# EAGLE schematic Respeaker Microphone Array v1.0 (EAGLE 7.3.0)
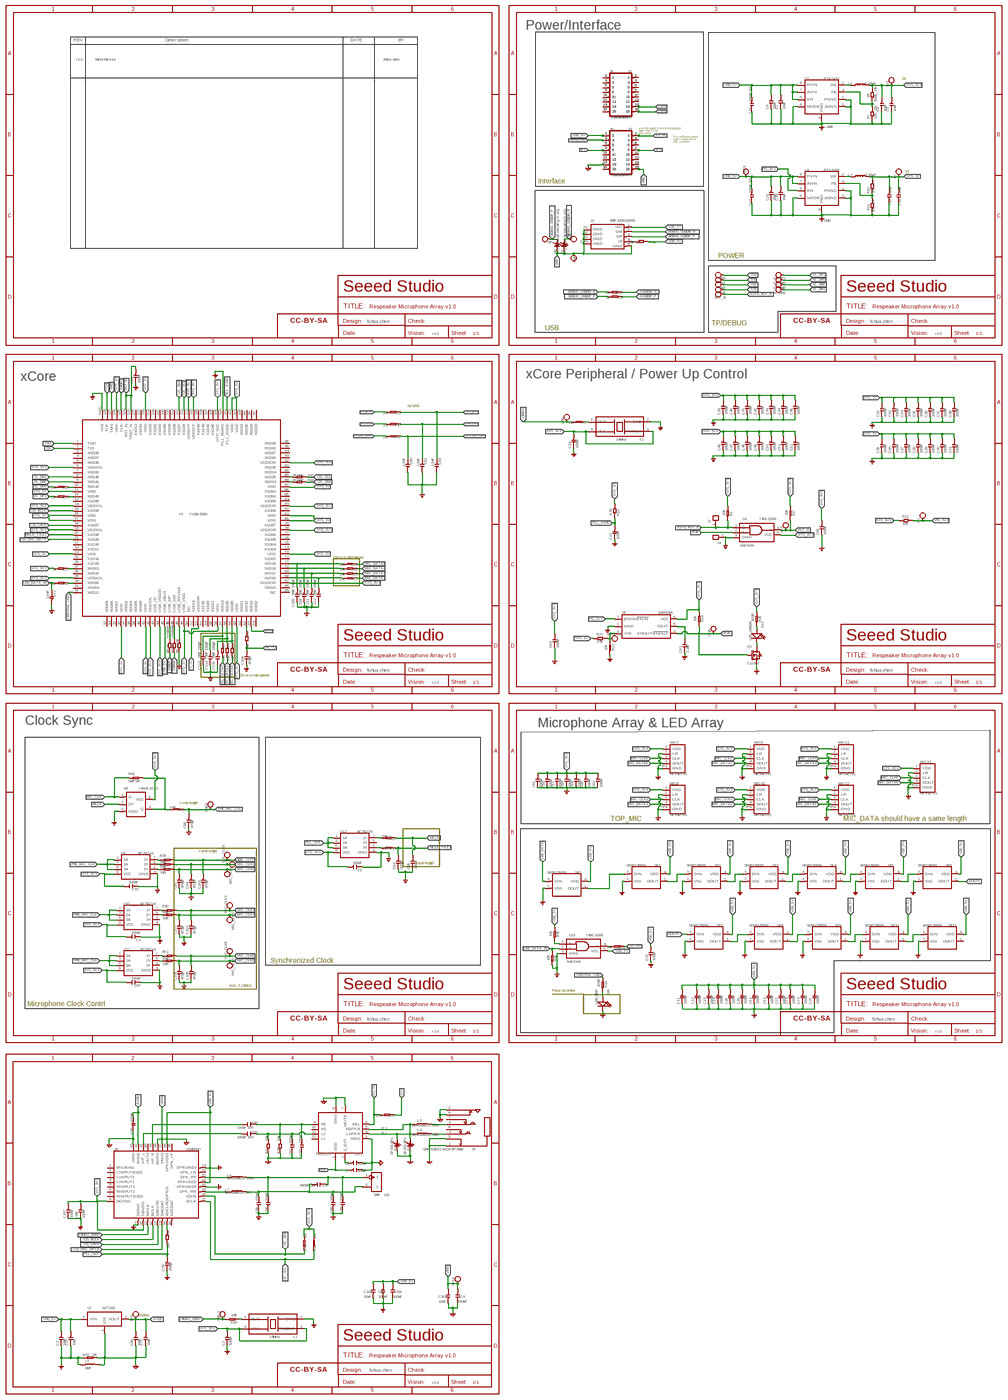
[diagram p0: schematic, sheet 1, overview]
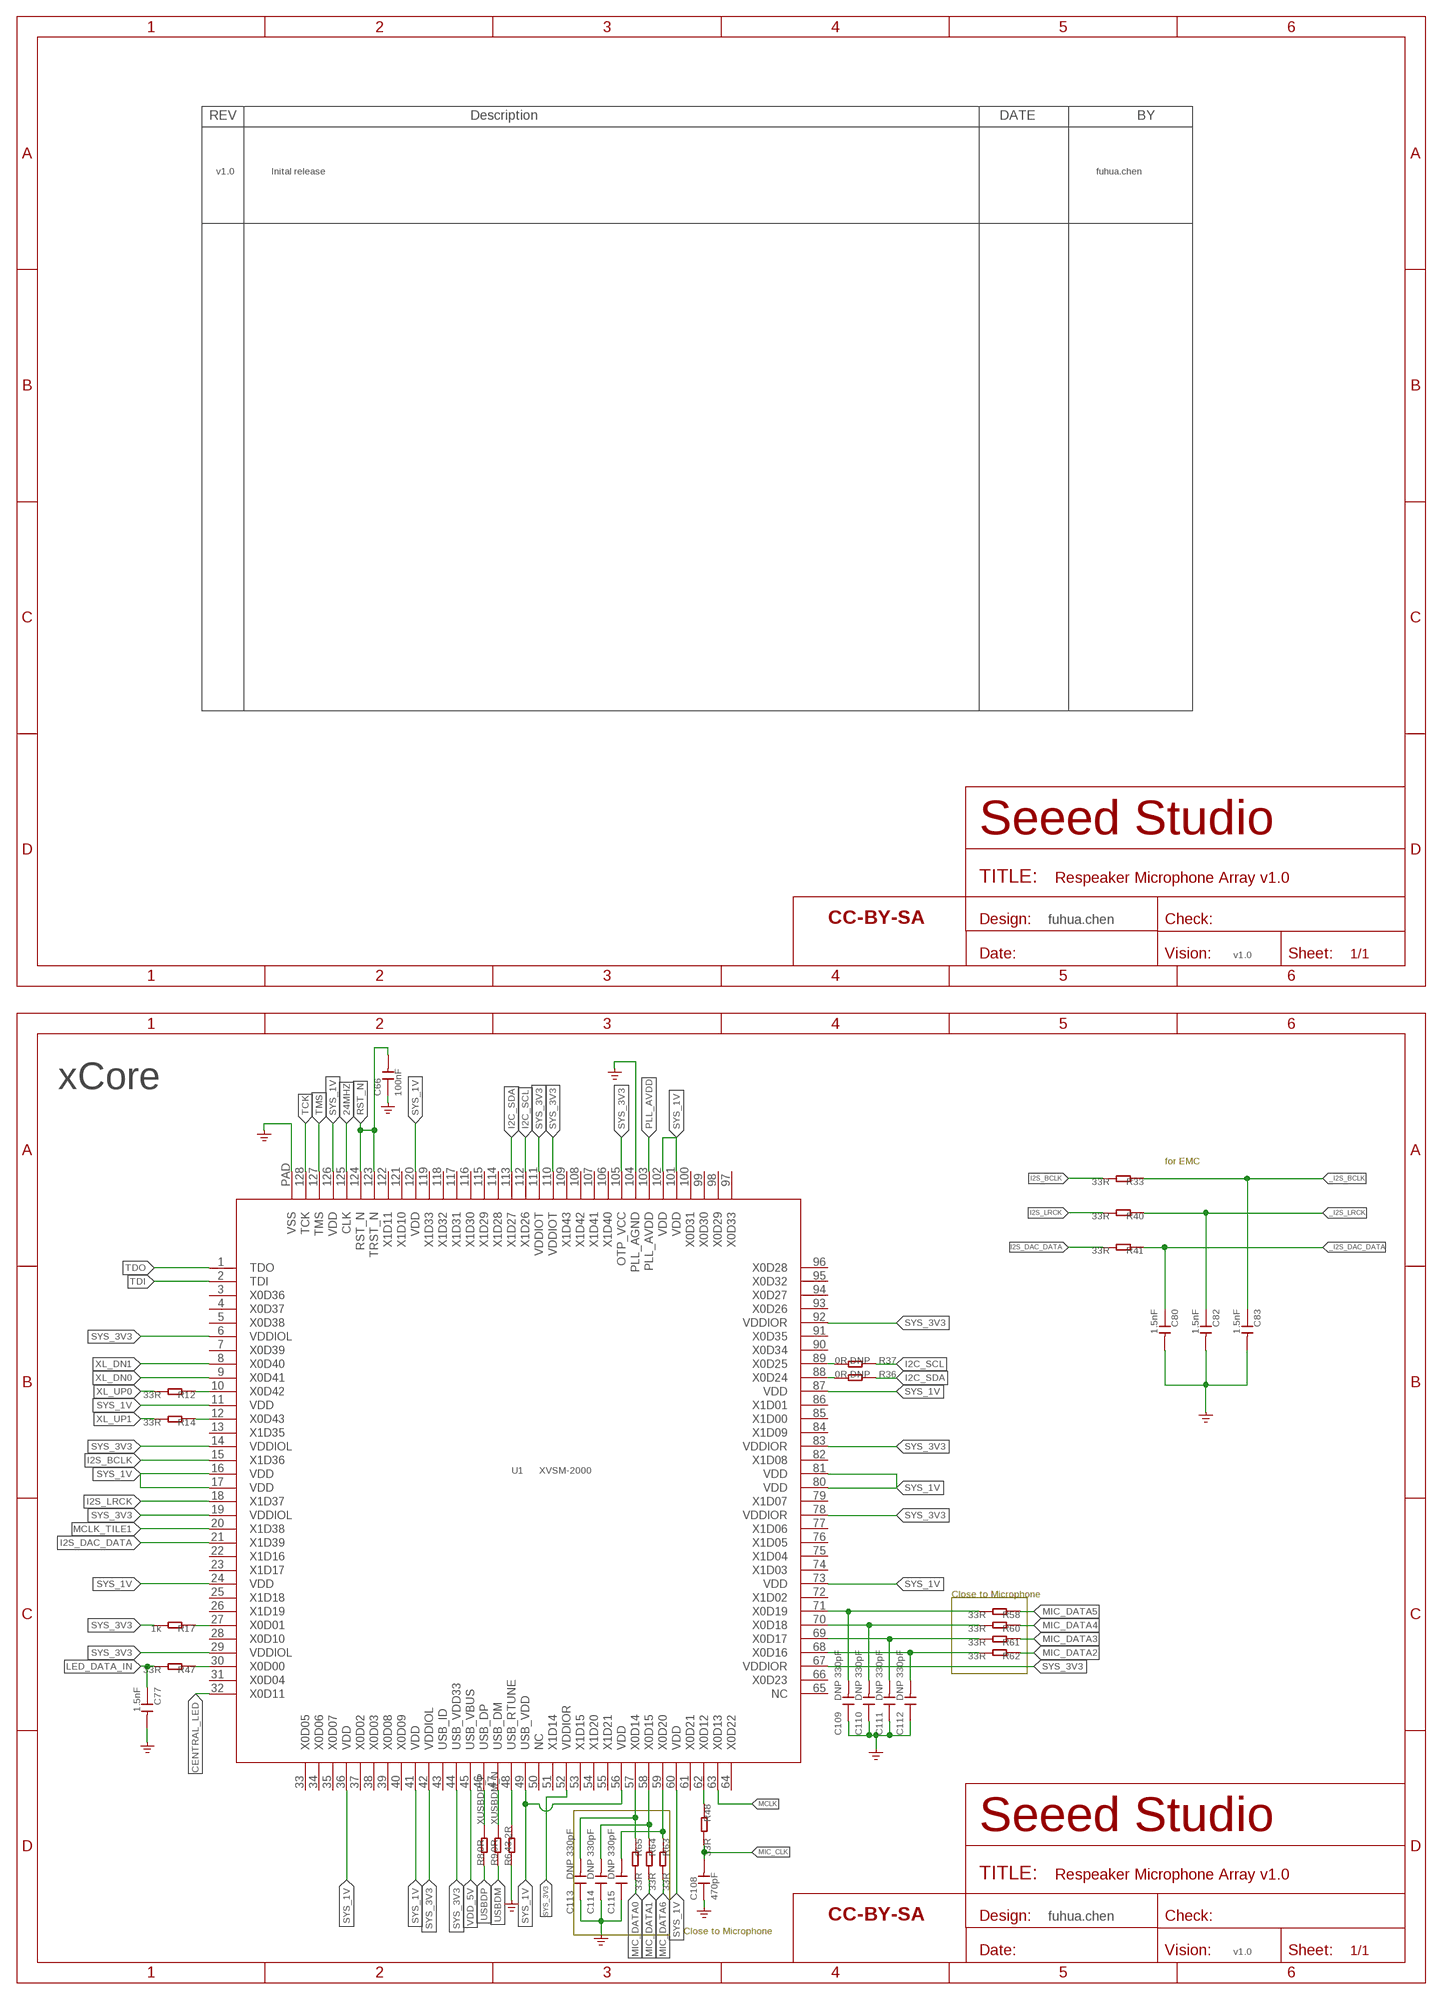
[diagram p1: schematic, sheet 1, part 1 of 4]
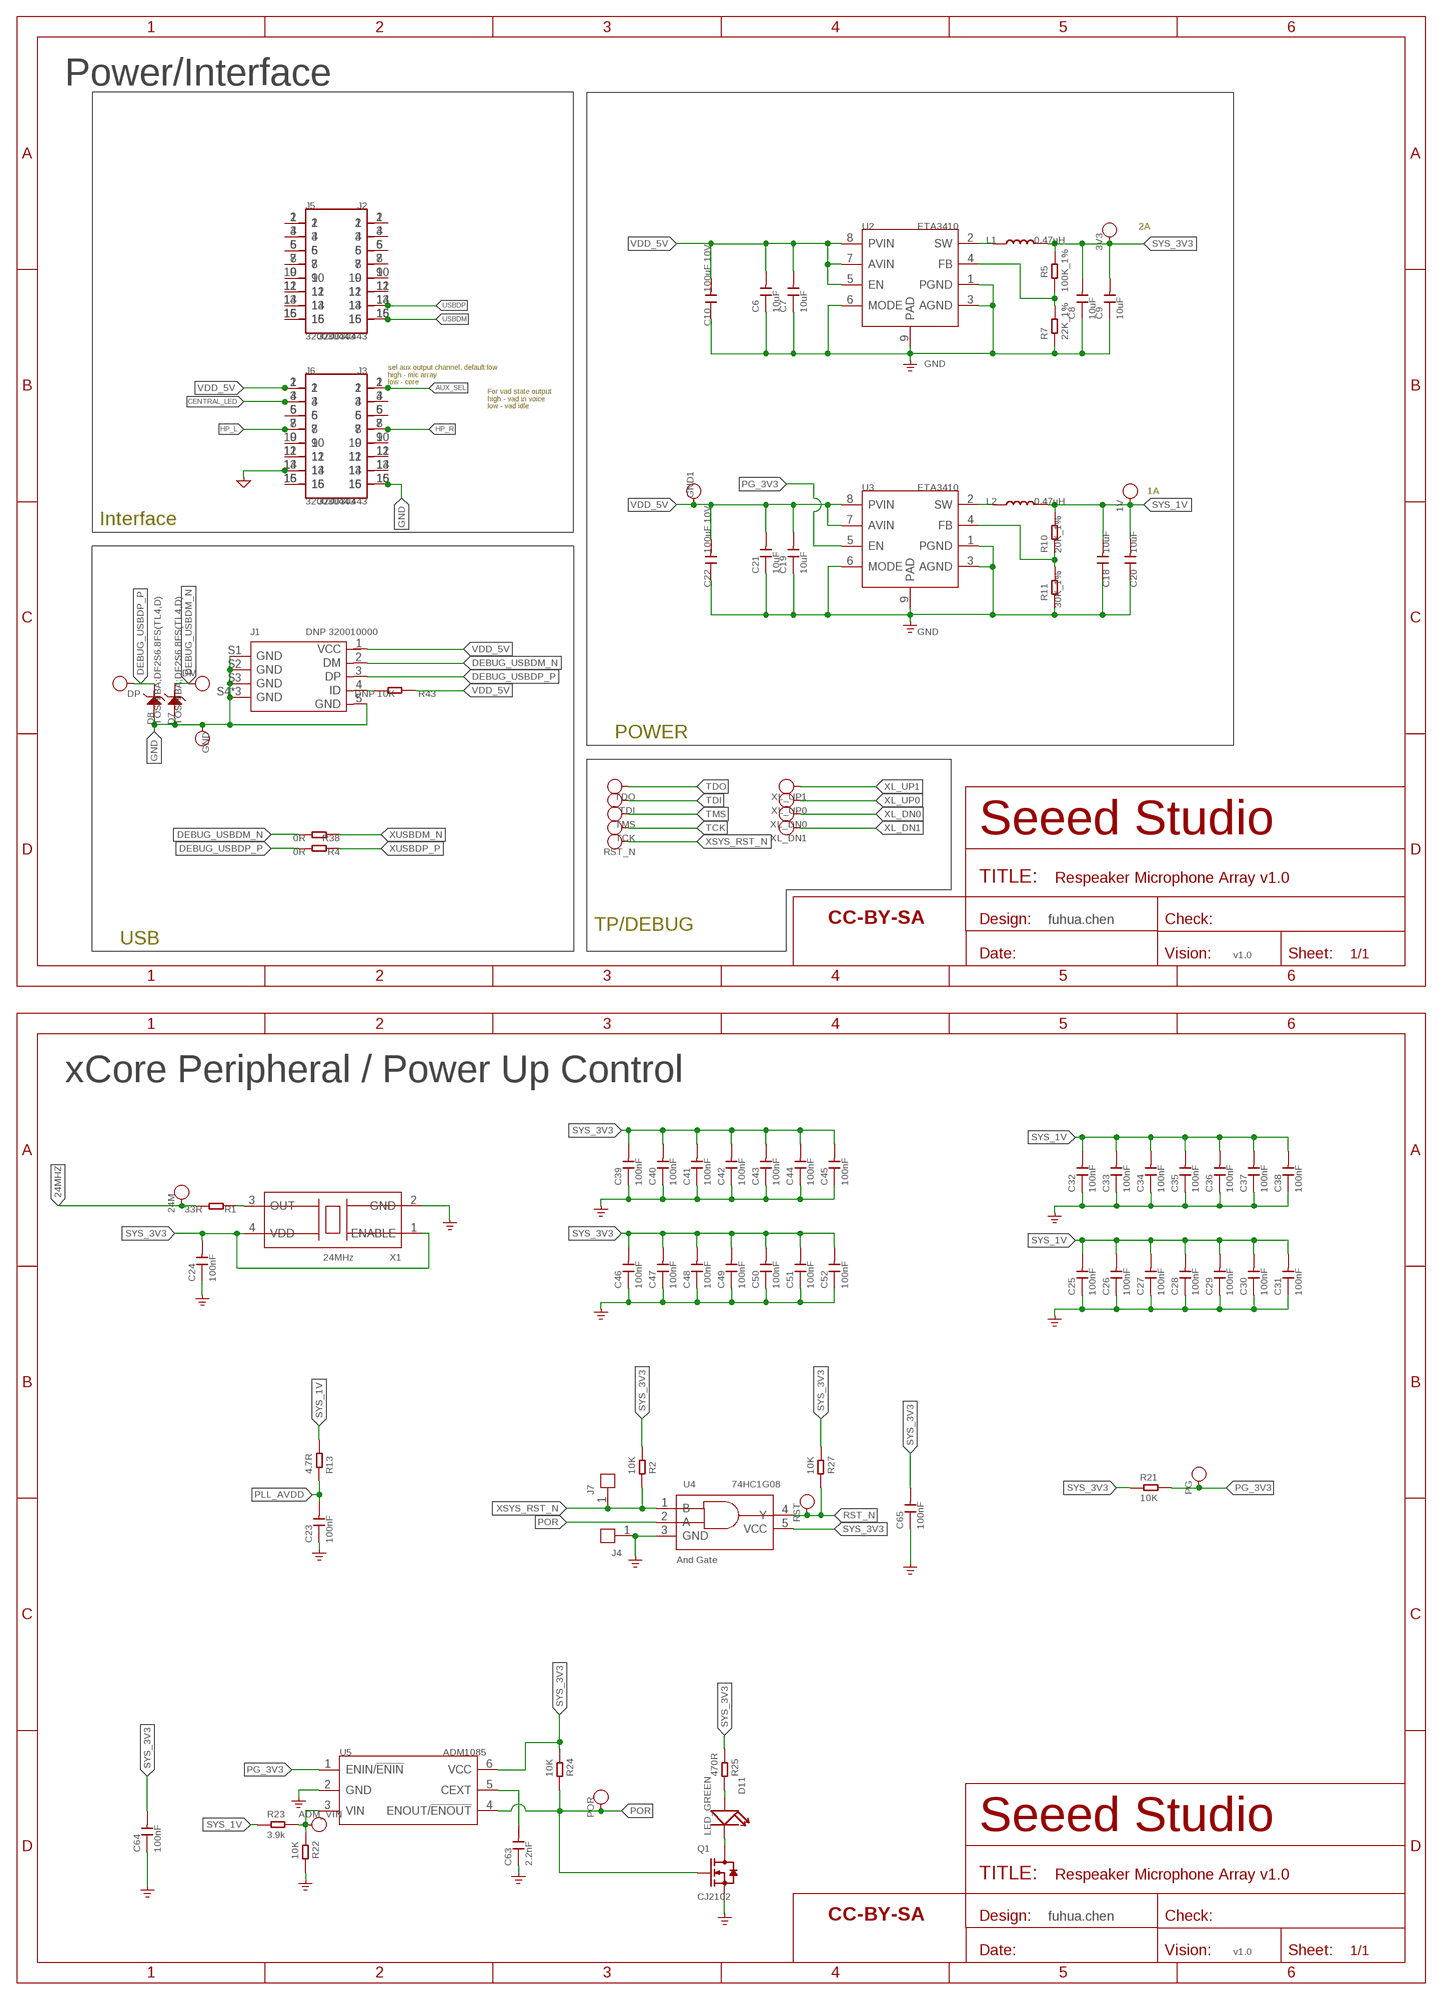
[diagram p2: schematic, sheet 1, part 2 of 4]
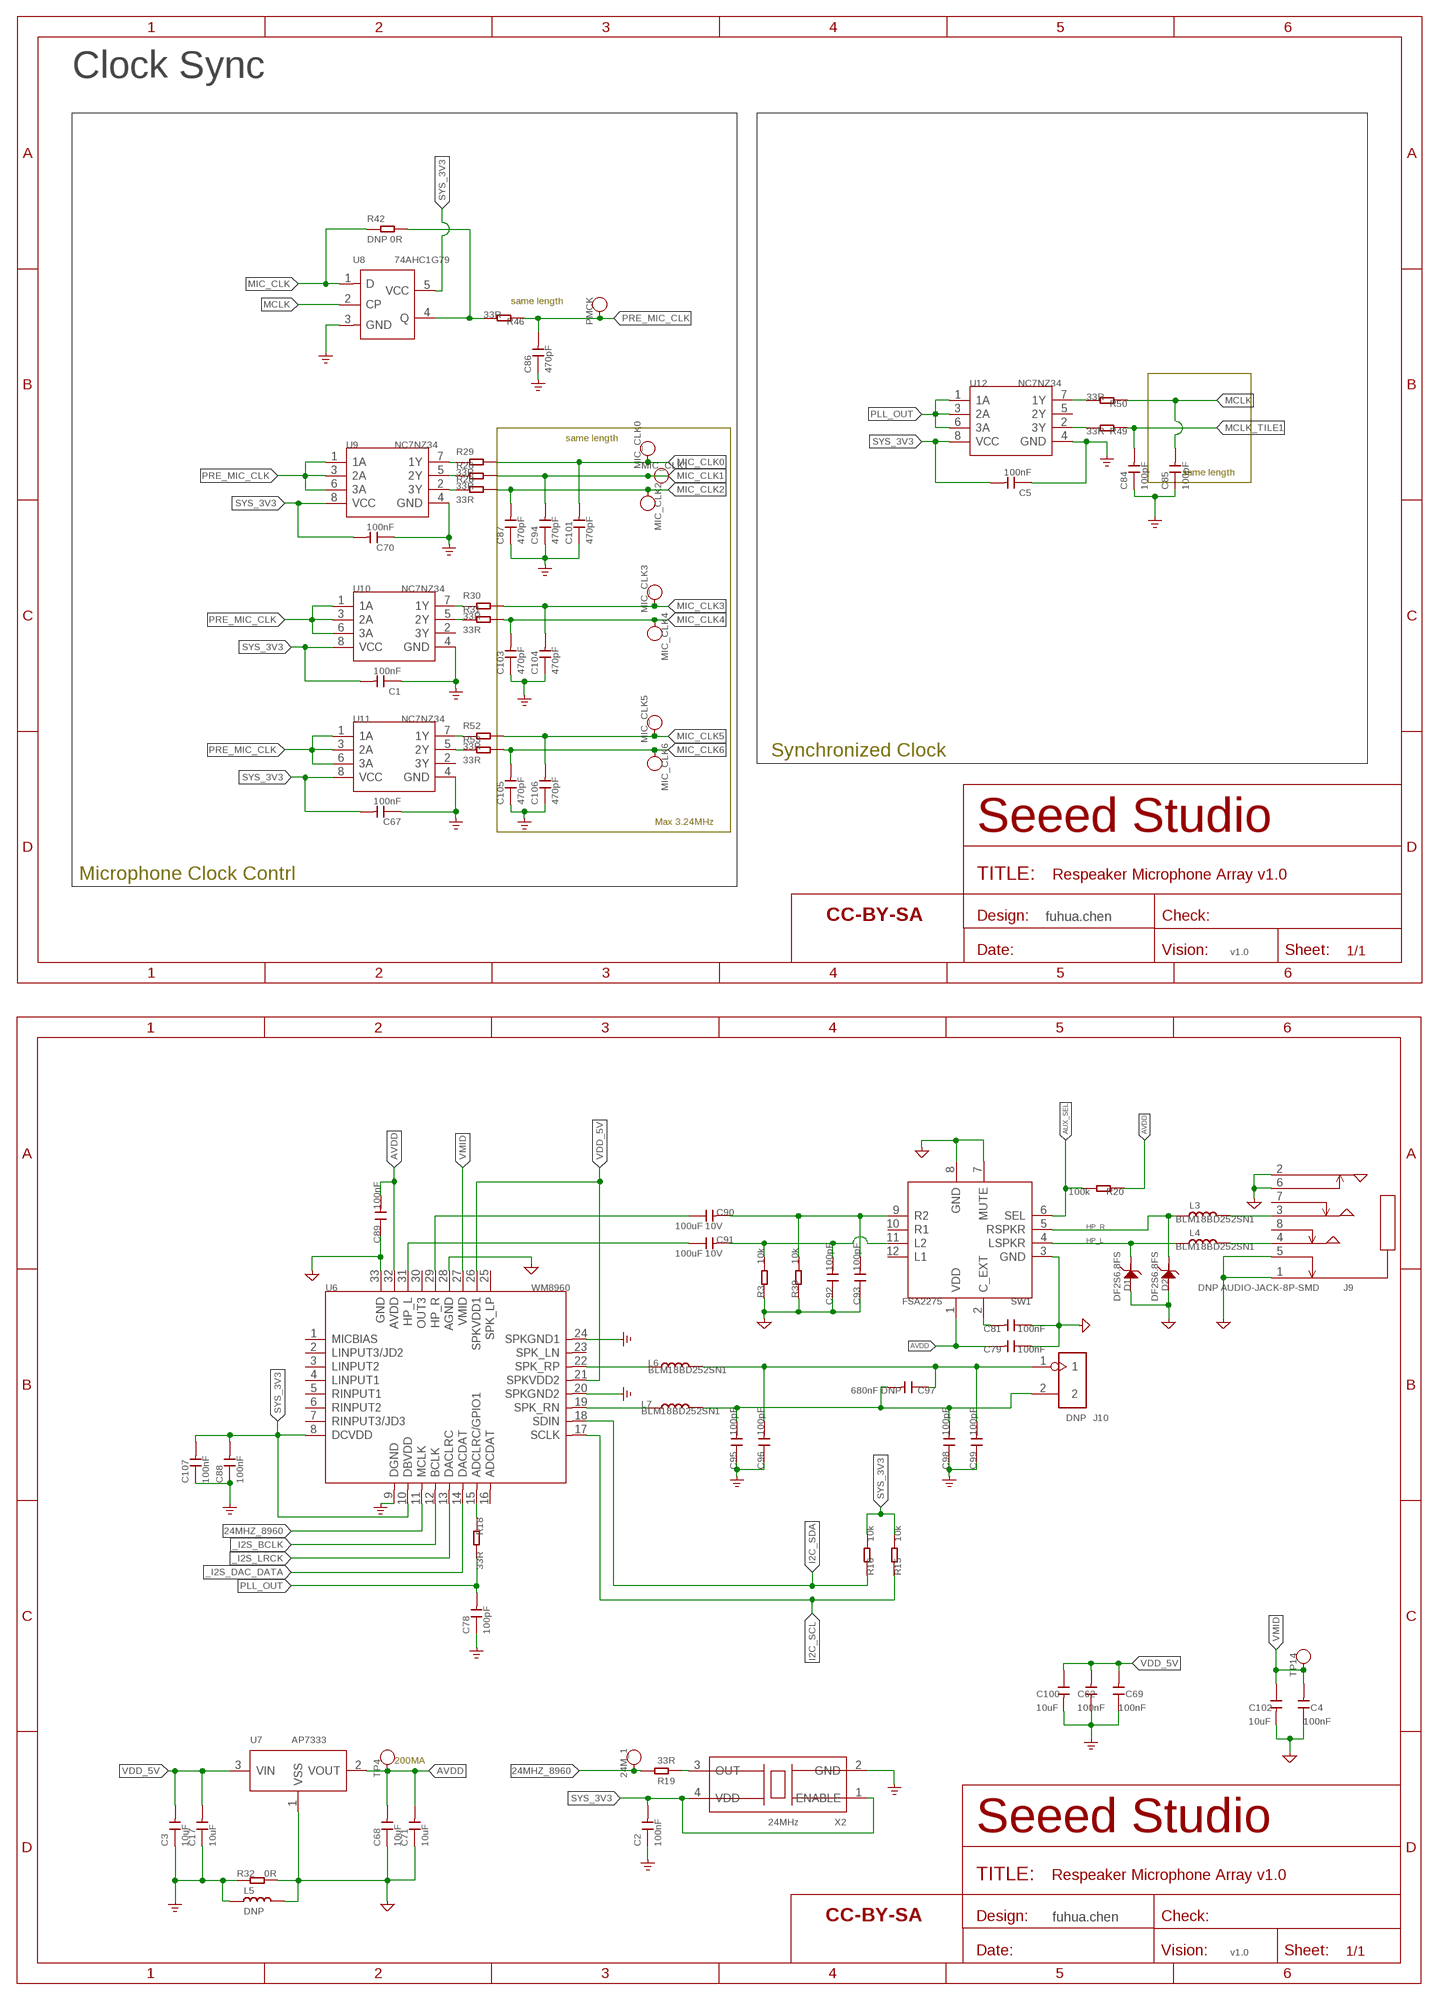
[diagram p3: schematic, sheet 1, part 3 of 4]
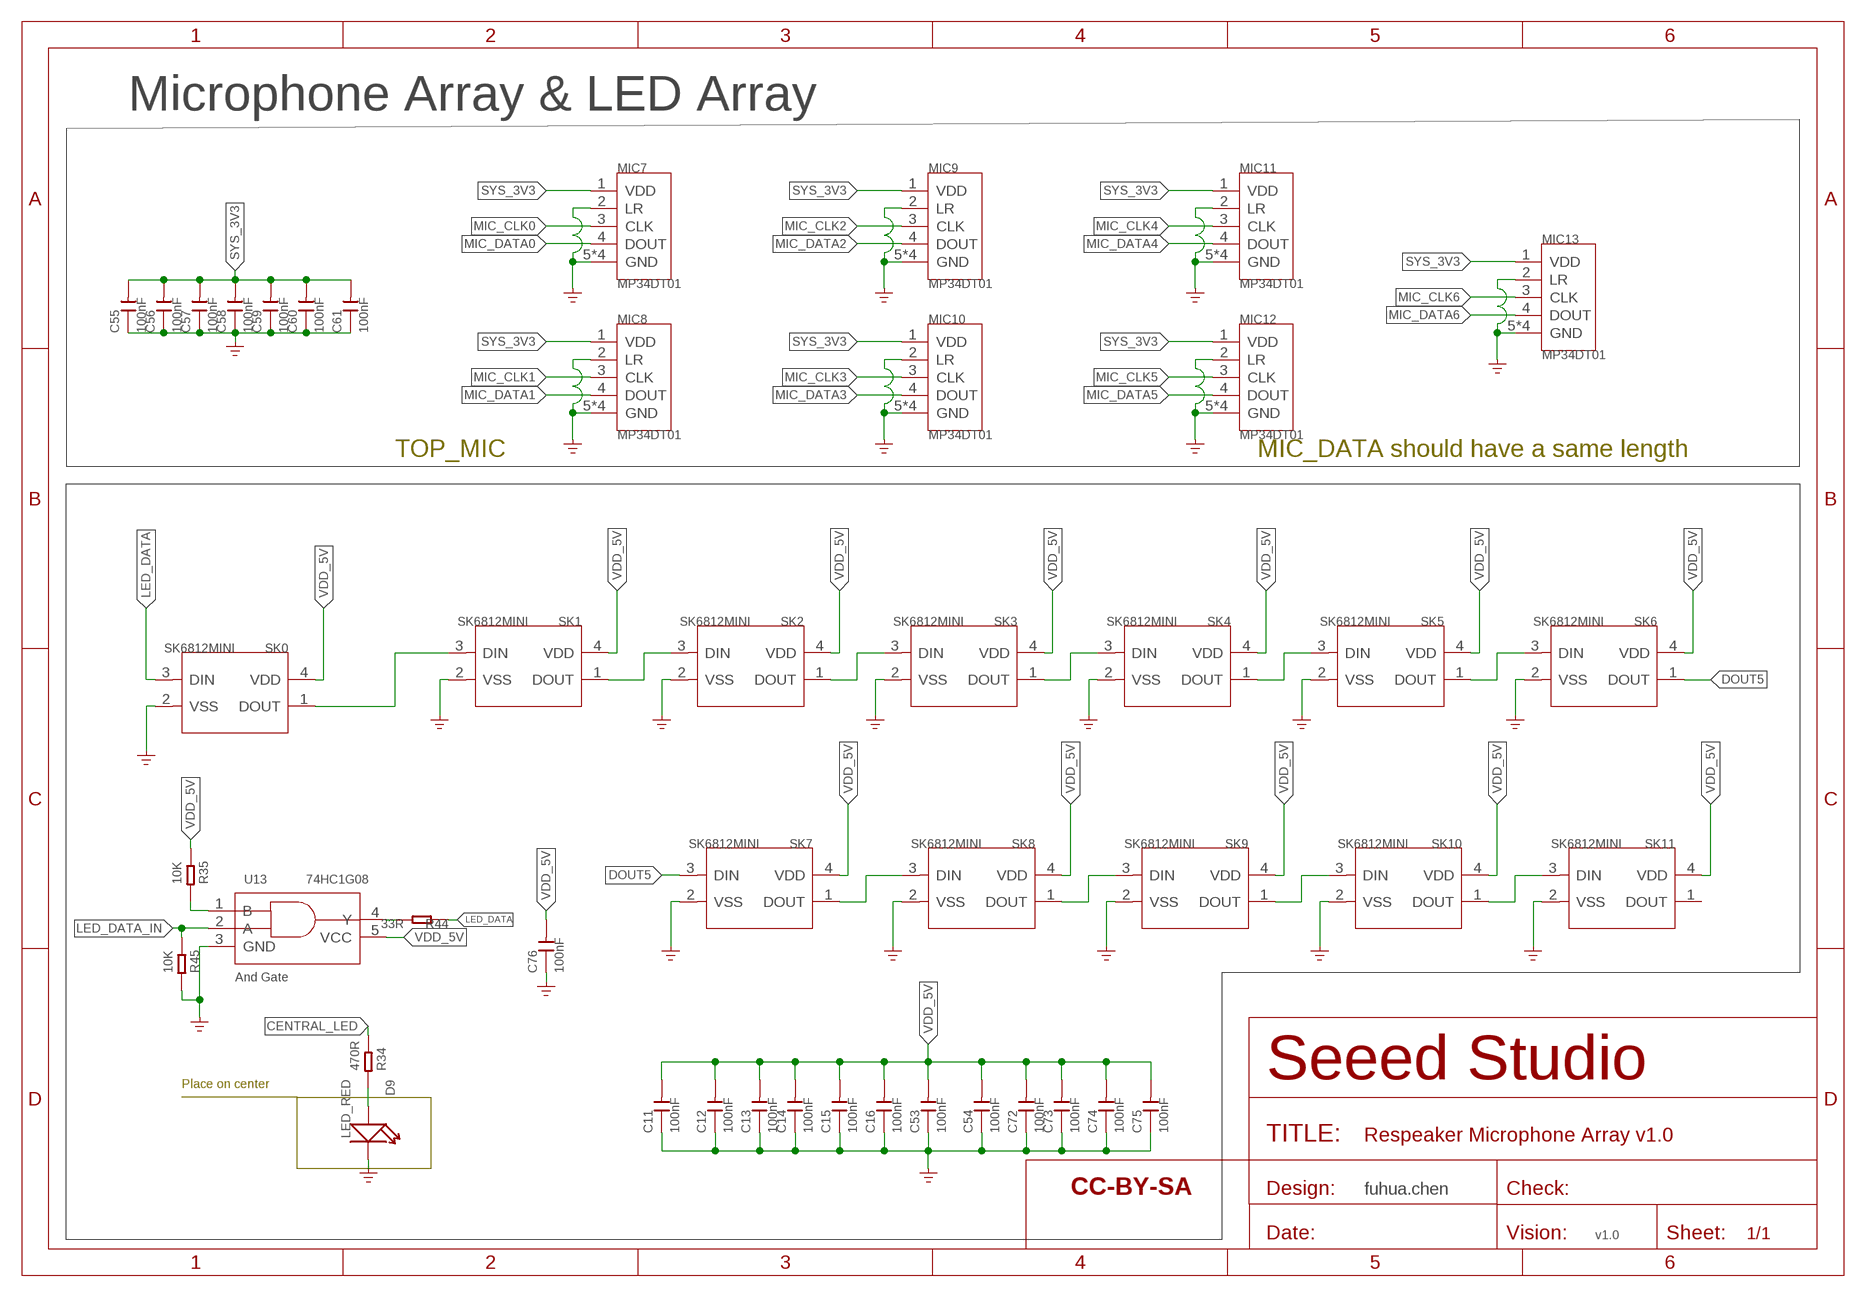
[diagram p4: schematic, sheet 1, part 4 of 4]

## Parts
1V  TEST-POINT'4545'  [TP-D45MIL]
3V3  TEST-POINT'4545'  [TP-D45MIL]
24M  TEST-POINT'4545'  [TP-D45MIL]
24M_1  TEST-POINT'4545'  [TP-D45MIL]
ADM_VIN  TEST-POINT'4545'  [TP-D45MIL]
C1  100nF  CAP-0402  [C0402]
C2  100nF  CAP-0402  [C0402]
C3  10uF  CAP-0603  [C0603]
C4  100nF  CAP-0402  [C0402]
C5  100nF  CAP-0402  [C0402]
C6  10uF  CAP-0603  [C0603]
C7  10uF  CAP-0603  [C0603]
C8  10uF  CAP-0603  [C0603]
C9  10uF  CAP-0603  [C0603]
C10  100uF 10V  CAP-1206  [C1206]
C11  100nF  CAP-0402  [C0402]
C12  100nF  CAP-0402  [C0402]
C13  100nF  CAP-0402  [C0402]
C14  100nF  CAP-0402  [C0402]
C15  100nF  CAP-0402  [C0402]
C16  100nF  CAP-0402  [C0402]
C17  10uF  CAP-0603  [C0603]
C18  10uF  CAP-0603  [C0603]
C19  10uF  CAP-0603  [C0603]
C20  10uF  CAP-0603  [C0603]
C21  10uF  CAP-0603  [C0603]
C22  100uF 10V  CAP-1206  [C1206]
C23  100nF  CAP-0402  [C0402]
C24  100nF  CAP-0402  [C0402]
C25  100nF  CAP-0402  [C0402]
C26  100nF  CAP-0402  [C0402]
C27  100nF  CAP-0402  [C0402]
C28  100nF  CAP-0402  [C0402]
C29  100nF  CAP-0402  [C0402]
C30  100nF  CAP-0402  [C0402]
C31  100nF  CAP-0402  [C0402]
C32  100nF  CAP-0402  [C0402]
C33  100nF  CAP-0402  [C0402]
C34  100nF  CAP-0402  [C0402]
C35  100nF  CAP-0402  [C0402]
C36  100nF  CAP-0402  [C0402]
C37  100nF  CAP-0402  [C0402]
C38  100nF  CAP-0402  [C0402]
C39  100nF  CAP-0402  [C0402]
C40  100nF  CAP-0402  [C0402]
C41  100nF  CAP-0402  [C0402]
C42  100nF  CAP-0402  [C0402]
C43  100nF  CAP-0402  [C0402]
C44  100nF  CAP-0402  [C0402]
C45  100nF  CAP-0402  [C0402]
C46  100nF  CAP-0402  [C0402]
C47  100nF  CAP-0402  [C0402]
C48  100nF  CAP-0402  [C0402]
C49  100nF  CAP-0402  [C0402]
C50  100nF  CAP-0402  [C0402]
C51  100nF  CAP-0402  [C0402]
C52  100nF  CAP-0402  [C0402]
C53  100nF  CAP-0402  [C0402]
C54  100nF  CAP-0402  [C0402]
C55  100nF  CAP-0402  [C0402]
C56  100nF  CAP-0402  [C0402]
C57  100nF  CAP-0402  [C0402]
C58  100nF  CAP-0402  [C0402]
C59  100nF  CAP-0402  [C0402]
C60  100nF  CAP-0402  [C0402]
C61  100nF  CAP-0402  [C0402]
C62  100nF  CAP-0402  [C0402]
C63  2.2nF  CAP-0402  [C0402]
C64  100nF  CAP-0402  [C0402]
C65  100nF  CAP-0402  [C0402]
C66  100nF  CAP-0402  [C0402]
C67  100nF  CAP-0402  [C0402]
C68  10uF  CAP-0603  [C0603]
C69  100nF  CAP-0402  [C0402]
C70  100nF  CAP-0402  [C0402]
C71  10uF  CAP-0603  [C0603]
C72  100nF  CAP-0402  [C0402]
C73  100nF  CAP-0402  [C0402]
C74  100nF  CAP-0402  [C0402]
C75  100nF  CAP-0402  [C0402]
C76  100nF  CAP-0402  [C0402]
C77  1.5nF  CAP-0402  [C0402]
C78  100pF  CAP-0402  [C0402]
C79  100nF  CAP-0402  [C0402]
C80  1.5nF  CAP-0402  [C0402]
C81  100nF  CAP-0402  [C0402]
C82  1.5nF  CAP-0402  [C0402]
C83  1.5nF  CAP-0402  [C0402]
C84  100pF  CAP-0402  [C0402]
C85  100pF  CAP-0402  [C0402]
C86  470pF  CAP-0402  [C0402]
C87  470pF  CAP-0402  [C0402]
C88  100nF  CAP-0402  [C0402]
C89  100nF  CAP-0402  [C0402]
C90  100uF 10V  CAP-1206  [C1206]
C91  100uF 10V  CAP-1206  [C1206]
C92  100pF  CAP-0402  [C0402]
C93  100pF  CAP-0402  [C0402]
C94  470pF  CAP-0402  [C0402]
C95  100pF  CAP-0402  [C0402]
C96  100pF  CAP-0402  [C0402]
C97  680nF DNP  CAP-0402  [C0402]
C98  100pF  CAP-0402  [C0402]
C99  100pF  CAP-0402  [C0402]
C100  10uF  CAP-0603  [C0603]
C101  470pF  CAP-0402  [C0402]
C102  10uF  CAP-0603  [C0603]
C103  470pF  CAP-0402  [C0402]
C104  470pF  CAP-0402  [C0402]
C105  470pF  CAP-0402  [C0402]
C106  470pF  CAP-0402  [C0402]
C107  100nF  CAP-0402  [C0402]
C108  470pF  CAP-0402  [C0402]
C109  DNP 330pF  CAP-0402  [C0402]
C110  DNP 330pF  CAP-0402  [C0402]
C111  DNP 330pF  CAP-0402  [C0402]
C112  DNP 330pF  CAP-0402  [C0402]
C113  DNP 330pF  CAP-0402  [C0402]
C114  DNP 330pF  CAP-0402  [C0402]
C115  DNP 330pF  CAP-0402  [C0402]
D1  DF2S6.8FS  D-ESD-2P'DF2S6.8FS'  [SOD-923]
D2  DF2S6.8FS  D-ESD-2P'DF2S6.8FS'  [SOD-923]
D7  TOSHIBA;DF2S6.8FS(TL4,D)  D-ESD-2P'DF2S6.8FS'  [SOD-923]
D8  TOSHIBA;DF2S6.8FS(TL4,D)  D-ESD-2P'DF2S6.8FS'  [SOD-923]
D9  LED_RED  LED-0402  [LED-0402]
D11  LED_GREEN  LED-0402  [LED-0402]
DM  TEST-POINT'4545'  [TP-D45MIL]
DP  TEST-POINT'4545'  [TP-D45MIL]
FR1  SEEEDSTUDIO-OPEN-SCH-FRAME  [SEEEDSTUDIO-PCB-FRAME]
FR2  SEEEDSTUDIO-OPEN-SCH-FRAME  [SEEEDSTUDIO-PCB-FRAME]
FR3  SEEEDSTUDIO-OPEN-SCH-FRAME  [SEEEDSTUDIO-PCB-FRAME]
FR4  SEEEDSTUDIO-OPEN-SCH-FRAME  [SEEEDSTUDIO-PCB-FRAME]
FR5  SEEEDSTUDIO-OPEN-SCH-FRAME  [SEEEDSTUDIO-PCB-FRAME]
FR7  SEEEDSTUDIO-OPEN-SCH-FRAME  [SEEEDSTUDIO-PCB-FRAME]
FR8  SEEEDSTUDIO-OPEN-SCH-FRAME  [SEEEDSTUDIO-PCB-FRAME]
GND  TEST-POINT'4545'  [TP-D45MIL]
GND1  TEST-POINT'4545'  [TP-D45MIL]
J1  DNP 320010000  MICRO-USB5+4P'5+4P'  [MICRO-USB5+4P-SMD-0.65-B]
J2  320030443  HEADER-2X8P-SMD-2.0  [H2X8-SMD-2.0]
J3  320030443  HEADER-2X8P-SMD-2.0  [H2X8-SMD-2.0]
J4  HEADER-1P'20'  [1P-40/25MIL]
J5  320030443  HEADER-2X8P-SMD-2.0  [H2X8-SMD-2.0]
J6  320030443  HEADER-2X8P-SMD-2.0  [H2X8-SMD-2.0]
J7  HEADER-1P'20'  [1P-40/25MIL]
J9  DNP AUDIO-JACK-8P-SMD  AUDIO-JACK-8P-SMD'PJ-393'  [AUDIO8P-SMD-3.5-14.5X6.1X4.0MM]
J10  DNP  HEADER-2P-65/35MIL  [H2-2.54]
L1  0.47uH  L-MPM201610SR33_T  [L201610]
L2  0.47uH  L-MPM201610SR33_T  [L201610]
L3  BLM18BD252SN1  INDUCTOR/FERRITE-BEAD'0603'  [L0603]
L4  BLM18BD252SN1  INDUCTOR/FERRITE-BEAD'0603'  [L0603]
L5  DNP  INDUCTOR/FERRITE-BEAD'0603'  [L0603]
L6  BLM18BD252SN1  INDUCTOR/FERRITE-BEAD'0603'  [L0603]
L7  BLM18BD252SN1  INDUCTOR/FERRITE-BEAD'0603'  [L0603]
MIC7  MP34DT01  MICROPHONE-MP34DT01  [HCLGA5P-3X4X1MM]
MIC8  MP34DT01  MICROPHONE-MP34DT01  [HCLGA5P-3X4X1MM]
MIC9  MP34DT01  MICROPHONE-MP34DT01  [HCLGA5P-3X4X1MM]
MIC10  MP34DT01  MICROPHONE-MP34DT01  [HCLGA5P-3X4X1MM]
MIC11  MP34DT01  MICROPHONE-MP34DT01  [HCLGA5P-3X4X1MM]
MIC12  MP34DT01  MICROPHONE-MP34DT01  [HCLGA5P-3X4X1MM]
MIC13  MP34DT01  MICROPHONE-MP34DT01  [HCLGA5P-3X4X1MM]
MIC_CLK0  TEST-POINT'4545'  [TP-D45MIL]
MIC_CLK1  TEST-POINT'4545'  [TP-D45MIL]
MIC_CLK2  TEST-POINT'4545'  [TP-D45MIL]
MIC_CLK3  TEST-POINT'4545'  [TP-D45MIL]
MIC_CLK4  TEST-POINT'4545'  [TP-D45MIL]
MIC_CLK5  TEST-POINT'4545'  [TP-D45MIL]
MIC_CLK6  TEST-POINT'4545'  [TP-D45MIL]
PG  TEST-POINT'4545'  [TP-D45MIL]
PMCK  TEST-POINT'4545'  [TP-D45MIL]
POR  TEST-POINT'4545'  [TP-D45MIL]
Q1  CJ2102  MOSFET-N+'SI1304BDL'  [SOT-323]
R1  33R  RES-0402  [R0402]
R2  10K  RES-0402  [R0402]
R3  10k  RES-0402  [R0402]
R4  0R  RES-0402  [R0402]
R5  100K_1%  RES-0402  [R0402]
R6  43.2R  RES-0402  [R0402]
R7  22K_1%  RES-0402  [R0402]
R8  0R  RES-0402  [R0402]
R9  0R  RES-0402  [R0402]
R10  20K_1%  RES-0402  [R0402]
R11  30K_1%  RES-0402  [R0402]
R12  33R  RES-0402  [R0402]
R13  4.7R  RES-0805  [R0805]
R14  33R  RES-0402  [R0402]
R15  10k  RES-0402  [R0402]
R16  10k  RES-0402  [R0402]
R17  1k  RES-0402  [R0402]
R18  33R  RES-0402  [R0402]
R19  33R  RES-0402  [R0402]
R20  100k  RES-0402  [R0402]
R21  10K  RES-0402  [R0402]
R22  10K  RES-0402  [R0402]
R23  3.9k  RES-0402  [R0402]
R24  10K  RES-0402  [R0402]
R25  470R  RES-0402  [R0402]
R26  33R  RES-0402  [R0402]
R27  10K  RES-0402  [R0402]
R28  33R  RES-0402  [R0402]
R29  33R  RES-0402  [R0402]
R30  33R  RES-0402  [R0402]
R31  33R  RES-0402  [R0402]
R32  0R  RES-0402  [R0402]
R33  33R  RES-0402  [R0402]
R34  470R  RES-0402  [R0402]
R35  10K  RES-0402  [R0402]
R36  0R DNP  RES-0402  [R0402]
R37  0R DNP  RES-0402  [R0402]
R38  0R  RES-0402  [R0402]
R39  10k  RES-0402  [R0402]
R40  33R  RES-0402  [R0402]
R41  33R  RES-0402  [R0402]
R42  DNP 0R  RES-0402  [R0402]
R43  DNP 10K  RES-0402  [R0402]
R44  33R  RES-0402  [R0402]
R45  10K  RES-0402  [R0402]
R46  33R  RES-0402  [R0402]
R47  33R  RES-0402  [R0402]
R48  33R  RES-0402  [R0402]
R49  33R  RES-0402  [R0402]
R50  33R  RES-0402  [R0402]
R52  33R  RES-0402  [R0402]
R53  33R  RES-0402  [R0402]
R58  33R  RES-0402  [R0402]
R60  33R  RES-0402  [R0402]
R61  33R  RES-0402  [R0402]
R62  33R  RES-0402  [R0402]
R63  33R  RES-0402  [R0402]
R64  33R  RES-0402  [R0402]
R65  33R  RES-0402  [R0402]
RST  TEST-POINT'4545'  [TP-D45MIL]
RST_N  TEST-POINT'4545'  [TP-D45MIL]
SK0  SK6812MINI  LED-RGB-4P-SK68122  [LED4-SMD-3.5X3.7MM]
SK1  SK6812MINI  LED-RGB-4P-SK68122  [LED4-SMD-3.5X3.7MM]
SK2  SK6812MINI  LED-RGB-4P-SK68122  [LED4-SMD-3.5X3.7MM]
SK3  SK6812MINI  LED-RGB-4P-SK68122  [LED4-SMD-3.5X3.7MM]
SK4  SK6812MINI  LED-RGB-4P-SK68122  [LED4-SMD-3.5X3.7MM]
SK5  SK6812MINI  LED-RGB-4P-SK68122  [LED4-SMD-3.5X3.7MM]
SK6  SK6812MINI  LED-RGB-4P-SK68122  [LED4-SMD-3.5X3.7MM]
SK7  SK6812MINI  LED-RGB-4P-SK68122  [LED4-SMD-3.5X3.7MM]
SK8  SK6812MINI  LED-RGB-4P-SK68122  [LED4-SMD-3.5X3.7MM]
SK9  SK6812MINI  LED-RGB-4P-SK68122  [LED4-SMD-3.5X3.7MM]
SK10  SK6812MINI  LED-RGB-4P-SK68122  [LED4-SMD-3.5X3.7MM]
SK11  SK6812MINI  LED-RGB-4P-SK68122  [LED4-SMD-3.5X3.7MM]
SW1  FSA2275  SWITCH-ANALOG-FSA2275  [LEAD12P-SMD-0.4-1.8X1.8X0.5MM]
TCK  TEST-POINT'4545'  [TP-D45MIL]
TDI  TEST-POINT'4545'  [TP-D45MIL]
TDO  TEST-POINT'4545'  [TP-D45MIL]
TMS  TEST-POINT'4545'  [TP-D45MIL]
TP4  TEST-POINT'4545'  [TP-D45MIL]
TP14  TEST-POINT'4545'  [TP-D45MIL]
U1  XVSM-2000  MCU-XUF216-512-TQ128  [TQFP128-0.4-14X14MM]
U2  ETA3410  CONVERTER-ETA3410  [DFN8G-0.5-2X2MM]
U3  ETA3410  CONVERTER-ETA3410  [DFN8G-0.5-2X2MM]
U4  74HC1G08  LOGIC-74HC1G08'GW'  [SOT-353]
U5  ADM1085  ANALOG-DEVICE-ADM1085  [SC-70-6]
U6  WM8960  AMPLIFIER-WM8960  [QFN32G-0.5-5X5MM]
U7  AP7333  PMIC-XC6206PMR  [SOT-23]
U8  74AHC1G79  LOGIC-74AHC/T1G79  [SOT-353]
U9  NC7NZ34  LOGIC-NC7NZ34  [US-8]
U10  NC7NZ34  LOGIC-NC7NZ34  [US-8]
U11  NC7NZ34  LOGIC-NC7NZ34  [US-8]
U12  NC7NZ34  LOGIC-NC7NZ34  [US-8]
U13  74HC1G08  LOGIC-74HC1G08'GW'  [SOT-353]
X1  24MHz  CRYSTAL-OSCILLATOR-NZ2520  [OSC-SMD-2.5X2.0X0.9MM]
X2  24MHz  CRYSTAL-OSCILLATOR-NZ2520  [OSC-SMD-2.5X2.0X0.9MM]
XL_DN0  TEST-POINT'4545'  [TP-D45MIL]
XL_DN1  TEST-POINT'4545'  [TP-D45MIL]
XL_UP0  TEST-POINT'4545'  [TP-D45MIL]
XL_UP1  TEST-POINT'4545'  [TP-D45MIL]

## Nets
24MHZ: 24M.T R1.2 U1.125(CLK)
24MHZ_8960: 24M_1.T R19.2 U6.11(MCLK)
$123: C90.1 U6.29(HP_R)
$124: C91.1 U6.31(HP_L)
_I2S_BCLK: C83.1 R33.1 U6.12(BCLK)
_I2S_DAC_DATA: C80.1 R41.1 U6.14(DACDAT)
_I2S_LRCK: C82.1 R40.1 U6.13(DACLRC)
AGND: C4.1 C68.1 C71.1 C79.1 C81.1 C89.1 C92.1 C93.1 C102.2 D1.2 D2.2 J3.14 J6.13 J9.1 J9.2 J9.5 J9.6 L5.2 R3.1 R32.2 R39.1 SW1.3(GND) SW1.7(MUTE) SW1.8(GND) U6.28(AGND) U6.33(GND) U7.1(VSS) ; supply symbol labelled GND_SIGNAL
AUX_SEL: J3.1 J6.2 R20.2 SW1.6(SEL)
AVDD: C68.2 C71.2 C79.2 C89.2 R20.1 SW1.1(VDD) TP4.T U6.32(AVDD) U7.2(VOUT)
CENTRAL_LED: J3.4 J6.3 R34.2 U1.32(X0D11)
DEBUG_USBDM_N: D7.1 DM.T J1.2(DM) R38.2
DEBUG_USBDP_P: D8.1 DP.T J1.3(DP) R4.2
DOUT5: SK6.1(DOUT) SK7.3(DIN)
GND: C1.1 C2.1 C3.1 C5.1 C6.1 C7.1 C8.1 C9.1 C10.1 C11.1 C12.1 C13.1 C14.1 C15.1 C16.1 C17.1 C18.1 C19.1 C20.1 C21.1 C22.1 C23.1 C24.1 C25.1 C26.1 C27.1 C28.1 C29.1 C30.1 C31.1 C32.1 C33.1 C34.1 C35.1 C36.1 C37.1 C38.1 C39.1 C40.1 C41.1 C42.1 C43.1 C44.1 C45.1 C46.1 C47.1 C48.1 C49.1 C50.1 C51.1 C52.1 C53.1 C54.1 C55.1 C56.1 C57.1 C58.1 C59.1 C60.1 C61.1 C62.1 C63.1 C64.1 C65.1 C66.1 C67.1 C69.1 C70.1 C72.1 C73.1 C74.1 C75.1 C76.1 C77.2 C78.1 C80.2 C82.2 C83.2 C84.1 C85.1 C86.1 C87.1 C88.1 C94.1 C95.1 C96.1 C98.1 C99.1 C100.2 C101.1 C103.1 C104.1 C105.1 C106.1 C107.1 C108.1 C109.1 C110.1 C111.1 C112.1 C113.1 C114.1 C115.1 D7.2 D8.2 D9.- GND.T J1.5(GND) J1.S1(GND) J1.S2(GND) J1.S3(GND) J1.S4(GND) J1.S5(GND) J1.S6(GND) J3.15 J4.1 J6.16 L5.1 MIC7.2(LR) MIC7.5(GND) MIC7.6(GND) MIC7.7(GND) MIC7.8(GND) MIC8.2(LR) MIC8.5(GND) MIC8.6(GND) MIC8.7(GND) MIC8.8(GND) MIC9.2(LR) MIC9.5(GND) MIC9.6(GND) MIC9.7(GND) MIC9.8(GND) MIC10.2(LR) MIC10.5(GND) MIC10.6(GND) MIC10.7(GND) MIC10.8(GND) MIC11.2(LR) MIC11.5(GND) MIC11.6(GND) MIC11.7(GND) MIC11.8(GND) MIC12.2(LR) MIC12.5(GND) MIC12.6(GND) MIC12.7(GND) MIC12.8(GND) MIC13.2(LR) MIC13.5(GND) MIC13.6(GND) MIC13.7(GND) MIC13.8(GND) Q1.2(S) R6.1 R7.1 R11.1 R22.1 R32.1 R45.1 SK0.2(VSS) SK1.2(VSS) SK2.2(VSS) SK3.2(VSS) SK4.2(VSS) SK5.2(VSS) SK6.2(VSS) SK7.2(VSS) SK8.2(VSS) SK9.2(VSS) SK10.2(VSS) SK11.2(VSS) U1.104(PLL_AGND) U1.PAD(VSS) U2.1(PGND) U2.3(AGND) U2.6(MODE) U2.9(PAD) U3.1(PGND) U3.3(AGND) U3.6(MODE) U3.9(PAD) U4.3(GND) U5.2(GND) U6.9(DGND) U6.20(SPKGND2) U6.24(SPKGND1) U8.3(GND) U9.4(GND) U10.4(GND) U11.4(GND) U12.4(GND) U13.3(GND) X1.2(GND) X2.2(GND) ; supply symbol labelled GND_POWER
HP_L: D1.1 J3.8 J6.7 L4.1 SW1.4(LSPKR)
HP_R: D2.1 J3.7 J6.8 L3.1 SW1.5(RSPKR)
I2C_SCL: R15.1 R37.1 U1.112(X1D26) U6.17(SCLK)
I2C_SDA: R16.1 R36.1 U1.113(X1D27) U6.18(SDIN)
I2S_BCLK: R33.2 U1.15(X1D36)
I2S_DAC_DATA: R41.2 U1.21(X1D39)
I2S_LRCK: R40.2 U1.18(X1D37)
LED_DATA: R44.1 SK0.3(DIN)
LED_DATA_IN: C77.1 R45.2 R47.2 U13.2(A)
MCLK: C85.2 R50.1 U1.63(X0D13) U8.2(CP)
MCLK_TILE1: C84.2 R49.1 U1.20(X1D38)
MIC_CLK: C108.2 R42.1 R48.2 U8.1(D)
MIC_CLK0: C101.2 MIC7.3(CLK) MIC_CLK0.T R29.2
MIC_CLK1: C94.2 MIC8.3(CLK) MIC_CLK1.T R26.2
MIC_CLK2: C87.2 MIC9.3(CLK) MIC_CLK2.T R28.2
MIC_CLK3: C104.2 MIC10.3(CLK) MIC_CLK3.T R30.2
MIC_CLK4: C103.2 MIC11.3(CLK) MIC_CLK4.T R31.2
MIC_CLK5: C106.2 MIC12.3(CLK) MIC_CLK5.T R52.2
MIC_CLK6: C105.2 MIC13.3(CLK) MIC_CLK6.T R53.2
MIC_DATA0: MIC7.4(DOUT) R65.2
MIC_DATA1: MIC8.4(DOUT) R64.2
MIC_DATA2: MIC9.4(DOUT) R62.1
MIC_DATA3: MIC10.4(DOUT) R61.1
MIC_DATA4: MIC11.4(DOUT) R60.1
MIC_DATA5: MIC12.4(DOUT) R58.1
MIC_DATA6: MIC13.4(DOUT) R63.2
N$1: R14.1 U1.12(X0D43)
N$2: R18.1 U6.15(ADCLRC/GPIO1)
N$3: L2.1 U3.2(SW)
N$4: R6.2 U1.48(USB_RTUNE)
N$5: R12.1 U1.10(X0D42)
N$6: R17.1 U1.27(X0D01)
N$7: ADM_VIN.T R22.2 R23.1 U5.3(VIN)
N$8: R10.1 R11.2 U3.4(FB)
N$9: D11.- Q1.3(D)
N$10: SK8.1(DOUT) SK9.3(DIN)
N$11: R1.1 X1.3(OUT)
N$12: D11.+ R25.1
N$13: SK1.1(DOUT) SK2.3(DIN)
N$14: C63.2 U5.5(CEXT)
N$15: R28.1 U9.2(3Y)
N$16: R53.1 U11.5(2Y)
N$17: SK2.1(DOUT) SK3.3(DIN)
N$18: C81.2 SW1.2(C_EXT)
N$19: SK3.1(DOUT) SK4.3(DIN)
N$20: SK4.1(DOUT) SK5.3(DIN)
N$21: R19.1 X2.3(OUT)
N$22: R26.1 U9.5(2Y)
N$23: R31.1 U10.5(2Y)
N$24: R29.1 U9.7(1Y)
N$25: R49.2 U12.2(3Y)
N$26: R50.2 U12.7(1Y)
N$27: J2.1 J5.2
N$28: R30.1 U10.7(1Y)
N$29: L1.1 U2.2(SW)
N$30: J2.2 J5.1
N$31: R47.1 U1.30(X0D00)
N$32: R5.1 R7.2 U2.4(FB)
N$33: R52.1 U11.7(1Y)
N$34: J2.3 J5.4
N$35: C109.2 R58.2 U1.71(X0D19)
N$36: C110.2 R60.2 U1.70(X0D18)
N$37: C111.2 R61.2 U1.69(X0D17)
N$38: C112.2 R62.2 U1.68(X0D16)
N$40: C115.2 R63.1 U1.59(X0D20)
N$41: C114.2 R64.1 U1.58(X0D15)
N$42: J3.5 J6.6
N$43: J1.4(ID) R43.2
N$44: SK5.1(DOUT) SK6.3(DIN)
N$45: SK7.1(DOUT) SK8.3(DIN)
N$46: R36.2 U1.88(X0D24)
N$47: SK9.1(DOUT) SK10.3(DIN)
N$48: SK10.1(DOUT) SK11.3(DIN)
N$49: SK0.1(DOUT) SK1.3(DIN)
N$50: D9.+ R34.1
N$51: J2.4 J5.3
N$52: J2.5 J5.6
N$53: R37.2 U1.89(X0D25)
N$54: C95.2 C97.2 C98.2 J10.2 L7.2
N$55: J9.3 L3.2
N$56: C90.2 C93.2 R39.2 SW1.9(R2)
N$57: J9.4 L4.2
N$58: J2.6 J5.5
N$59: J2.7 J5.8
N$60: J2.8 J5.7
N$61: C91.2 C92.2 R3.2 SW1.11(L2)
N$62: L6.1 U6.22(SPK_RP)
N$63: J2.9 J5.10
N$64: J2.10 J5.9
N$65: L7.1 U6.19(SPK_RN)
N$66: C96.2 C97.1 C99.2 J10.1 L6.2
N$67: J2.11 J5.12
N$68: J2.12 J5.11
N$69: J2.14 J5.13
N$70: J2.16 J5.15
N$71: R44.2 U13.4(Y)
N$72: R35.1 U13.1(B)
N$73: J3.6 J6.5
N$74: J3.9 J6.10
N$75: J3.10 J6.9
N$76: J3.11 J6.12
N$77: J3.12 J6.11
N$78: J3.13 J6.14
N$79: J3.16 J6.15
N$80: R42.2 R46.2 U8.4(Q)
N$81: R48.1 U1.62(X0D12)
N$82: C113.2 R65.1 U1.57(X0D14)
N$83: J3.3 J6.4
PG_3V3: PG.T R21.1 U3.5(EN) U5.1(ENIN/!ENIN)
PLL_AVDD: C23.2 R13.1 U1.103(PLL_AVDD)
PLL_OUT: C78.2 R18.2 U12.1(1A) U12.3(2A) U12.6(3A)
POR: POR.T Q1.1(G) R24.1 U4.2(A) U5.4(ENOUT/!ENOUT)
PRE_MIC_CLK: C86.2 PMCK.T R46.1 U9.1(1A) U9.3(2A) U9.6(3A) U10.1(1A) U10.3(2A) U10.6(3A) U11.1(1A) U11.3(2A) U11.6(3A)
RST_N: C66.2 R27.1 RST.T U1.123(TRST_N) U1.124(RST_N) U4.4(Y)
SYS_1V: 1V.T C18.2 C20.2 C25.2 C26.2 C27.2 C28.2 C29.2 C30.2 C31.2 C32.2 C33.2 C34.2 C35.2 C36.2 C37.2 C38.2 L2.2 R10.2 R13.2 R23.2 U1.11(VDD) U1.16(VDD) U1.17(VDD) U1.24(VDD) U1.36(VDD) U1.41(VDD) U1.49(USB_VDD) U1.56(VDD) U1.60(VDD) U1.73(VDD) U1.80(VDD) U1.81(VDD) U1.87(VDD) U1.101(VDD) U1.102(VDD) U1.120(VDD) U1.126(VDD)
SYS_3V3: 3V3.T C1.2 C2.2 C5.2 C8.2 C9.2 C24.2 C39.2 C40.2 C41.2 C42.2 C43.2 C44.2 C45.2 C46.2 C47.2 C48.2 C49.2 C50.2 C51.2 C52.2 C55.2 C56.2 C57.2 C58.2 C59.2 C60.2 C61.2 C64.2 C65.2 C67.2 C70.2 C88.2 C107.2 L1.2 MIC7.1(VDD) MIC8.1(VDD) MIC9.1(VDD) MIC10.1(VDD) MIC11.1(VDD) MIC12.1(VDD) MIC13.1(VDD) R2.2 R5.2 R15.2 R16.2 R17.2 R21.2 R24.2 R25.2 R27.2 U1.6(VDDIOL) U1.14(VDDIOL) U1.19(VDDIOL) U1.29(VDDIOL) U1.42(VDDIOL) U1.44(USB_VDD33) U1.52(VDDIOR) U1.67(VDDIOR) U1.78(VDDIOR) U1.83(VDDIOR) U1.92(VDDIOR) U1.105(OTP_VCC) U1.110(VDDIOT) U1.111(VDDIOT) U4.5(VCC) U5.6(VCC) U6.8(DCVDD) U6.10(DBVDD) U8.5(VCC) U9.8(VCC) U10.8(VCC) U11.8(VCC) U12.8(VCC) X1.1(ENABLE) X1.4(VDD) X2.1(ENABLE) X2.4(VDD)
TCK: TCK.T U1.128(TCK)
TDI: TDI.T U1.2(TDI)
TDO: TDO.T U1.1(TDO)
TMS: TMS.T U1.127(TMS)
USBDM: J2.15 J5.16 R9.1
USBDP: J2.13 J5.14 R8.1
VDD_5V: C3.2 C6.2 C7.2 C10.2 C11.2 C12.2 C13.2 C14.2 C15.2 C16.2 C17.2 C19.2 C21.2 C22.2 C53.2 C54.2 C62.2 C69.2 C72.2 C73.2 C74.2 C75.2 C76.2 C100.1 GND1.T J1.1(VCC) J3.2 J6.1 R35.2 R43.1 SK0.4(VDD) SK1.4(VDD) SK2.4(VDD) SK3.4(VDD) SK4.4(VDD) SK5.4(VDD) SK6.4(VDD) SK7.4(VDD) SK8.4(VDD) SK9.4(VDD) SK10.4(VDD) SK11.4(VDD) U1.45(USB_VBUS) U2.5(EN) U2.7(AVIN) U2.8(PVIN) U3.7(AVIN) U3.8(PVIN) U6.21(SPKVDD2) U6.26(SPKVDD1) U7.3(VIN) U13.5(VCC)
VMID: C4.2 C102.1 TP14.T U6.27(VMID)
XL_DN0: U1.9(X0D41) XL_DN0.T
XL_DN1: U1.8(X0D40) XL_DN1.T
XL_UP0: R12.2 XL_UP0.T
XL_UP1: R14.2 XL_UP1.T
XSYS_RST_N: J7.1 R2.1 RST_N.T U4.1(B)
XUSBDM_N: R9.2 R38.1 U1.47(USB_DM)
XUSBDP_P: R4.1 R8.2 U1.46(USB_DP)
Unconnected: J9.7 J9.8 SK11.1(DOUT) SW1.10(R1) SW1.12(L1) U1.3(X0D36) U1.4(X0D37) U1.5(X0D38) U1.7(X0D39) U1.13(X1D35) U1.22(X1D16) U1.23(X1D17) U1.25(X1D18) U1.26(X1D19) U1.28(X0D10) U1.31(X0D04) U1.33(X0D05) U1.34(X0D06) U1.35(X0D07) U1.37(X0D02) U1.38(X0D03) U1.39(X0D08) U1.40(X0D09) U1.43(USB_ID) U1.50(NC) U1.51(X1D14) U1.53(X1D15) U1.54(X1D20) U1.55(X1D21) U1.61(X0D21) U1.64(X0D22) U1.65(NC) U1.66(X0D23) U1.72(X1D02) U1.74(X1D03) U1.75(X1D04) U1.76(X1D05) U1.77(X1D06) U1.79(X1D07) U1.82(X1D08) U1.84(X1D09) U1.85(X1D00) U1.86(X1D01) U1.90(X0D34) U1.91(X0D35) U1.93(X0D26) U1.94(X0D27) U1.95(X0D32) U1.96(X0D28) U1.97(X0D33) U1.98(X0D29) U1.99(X0D30) U1.100(X0D31) U1.106(X1D40) U1.107(X1D41) U1.108(X1D42) U1.109(X1D43) U1.114(X1D28) U1.115(X1D29) U1.116(X1D30) U1.117(X1D31) U1.118(X1D32) U1.119(X1D33) U1.121(X1D10) U1.122(X1D11) U6.1(MICBIAS) U6.2(LINPUT3/JD2) U6.3(LINPUT2) U6.4(LINPUT1) U6.5(RINPUT1) U6.6(RINPUT2) U6.7(RINPUT3/JD3) U6.16(ADCDAT) U6.23(SPK_LN) U6.25(SPK_LP) U6.30(OUT3) U10.2(3Y) U11.2(3Y) U12.5(2Y)

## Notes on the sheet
- Power/Interface
- v1.0 | Inital release | fuhua.chen
- 2A
- sel aux output channel. default:low
  high - mic array
  low - core
- For vad state output
  high - vad in voice
  low - vad idle
- 1A
- Interface
- POWER
- fuhua.chen | fuhua.chen
- TP/DEBUG
- USB
- v1.0 | v1.0
- xCore | xCore Peripheral / Power Up Control
- for EMC
- And Gate
- Close to Microphone
- fuhua.chen | fuhua.chen
- Close to Microphone
- v1.0 | v1.0
- Clock Sync | Microphone Array & LED Array
- same length
- TOP_MIC | MIC_DATA should have a same length
- same length
- same length
- Synchronized Clock | And Gate
- Max 3.24MHz
- Place on center
- Microphone Clock Contrl
- fuhua.chen | fuhua.chen
- v1.0 | v1.0
- 200MA
- fuhua.chen
- v1.0

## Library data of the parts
1V 3V3 24M 24M_1 ADM_VIN DM DP GND GND1 MIC_CLK0 MIC_CLK1-MIC_CLK6 PG PMCK POR RST RST_N TCK TDI TDO TMS TP4 TP14 XL_DN0 XL_DN1 XL_UP0 XL_UP1 = Discrete-new:TEST-POINT; PARTNO: DNP
C1-C115 = Discrete-new:CAP: Ceramic Capacitors
D1 D2 D7 D8 = Discrete-new:D-ESD-2P: SOD-923:304060009;SOD-123:304060001
D9 D11 = Discrete-new:LED
FR1-FR5 FR7 FR8 = moudle-new:SEEEDSTUDIO-OPEN-SCH-FRAME
J1 = Connector-new:MICRO-USB5+4P: 5+4P-SMD-0.65-B:320010000;5+2P-SMD-0.65-AB:340032001
J2 J3 J5 J6 = Connector-new:HEADER-2X8P
J4 J7 = Connector-new:HEADER-1P
J9 = Connector-new:AUDIO-JACK-8P-SMD: 320040009
J10 = Connector-new:HEADER-2P
L1 L2 = Discrete-new:L
L3-L7 = Discrete-new:INDUCTOR/FERRITE-BEAD
MIC7-MIC13 = Discrete-new:MICROPHONE-MP34DT01
Q1 = Discrete-new:MOSFET-N+: IRLL014: http://www.vishay.com/docs/91319/sihll014.pdf
R1-R25 R27 R32-R41 R43-R50 R58 R60-R65 = Discrete-new:RES
R26 R28-R31 R42 R52 R53 = C-R-package test:RES
SK0 SK1-SK11 = Discrete-new:LED-RGB-4P: 304990003
SW1 = template:SWITCH-ANALOG-FSA2275
U1 = IC-new:MCU-XUF216-512-TQ128
U2 U3 = IC-new:CONVERTER-ETA3410: 3MHZ 2A High Step-Down Converter in DFN2x2-8L Package
U4 U13 = IC-new:LOGIC-74HC1G08: 2-input AND gate
U5 = IC-new:ANALOG-DEVICE-ADM1085
U6 = IC-new:AMPLIFIER-WM8960
U7 = IC-new:PMIC-XC6206P: LOW ESR Cap.Compatible Positive Voltage Regulators
U8 = IC-new:LOGIC-74AHC/T1G79
U9-U12 = IC-new:LOGIC-NC7NZ34
X1 X2 = Discrete-new:CRYSTAL-OSCILLATOR

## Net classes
0 default: width 0.025 mm, drill 0.203 mm, clearance 0.102 mm

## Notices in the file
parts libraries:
moudle-new: This work is licensed under the Creative Commons Attribution 4.0 International License.
To view a copy of this license,visit:
http://creativecommons.org/licenses/by-sa/4.0
moudle-new: CC-BY-SA
